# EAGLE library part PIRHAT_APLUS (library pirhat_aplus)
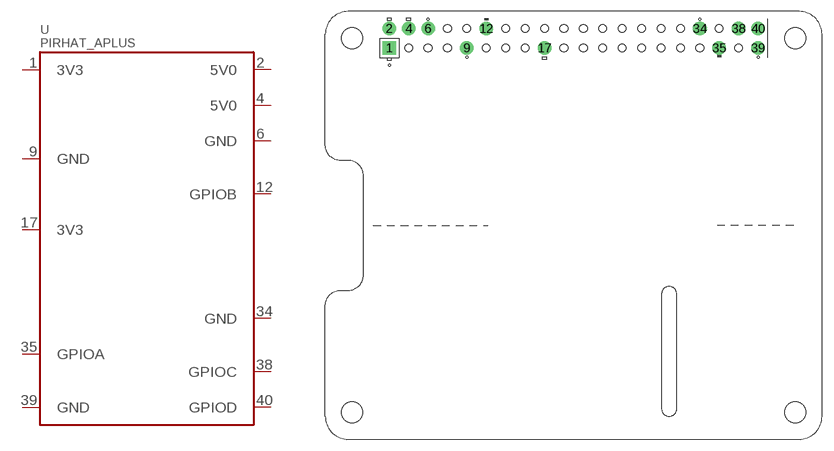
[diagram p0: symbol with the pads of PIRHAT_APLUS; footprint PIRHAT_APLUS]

Designator prefix -

## PIRHAT_APLUS  [PIRHAT_APLUS]
1  3V3  pwr
2  5V0  pwr
4  5V0  pwr
6  GND  sup
9  GND  sup
12  GPIOB
17  3V3  pwr
34  GND  sup
35  GPIOA
38  GPIOC
39  GND  sup
40  GPIOD

## Footprint PIRHAT_APLUS (pad centres in mm)
Raspberry Pi Zero W IR Hat, full outline with position of big connectors & drill holes
drill 1 pad 1.778 square: 1 8.37,51.235
drill 1 pad 1.778: 2 8.37,53.775; 4 10.91,53.775; 6 13.45,53.775; 9 18.53,51.235; 12 21.07,53.775; 17 28.69,51.235; 34 49.01,53.775; 35 51.55,51.235; 38 54.09,53.775; 39 56.63,51.235; 40 56.63,53.775
hole 1 at 54.09,51.235
hole 1 at 51.55,53.775
hole 1 at 31.23,51.235
hole 1 at 26.15,51.235
hole 1 at 15.99,53.775
hole 1 at 49.01,51.235
hole 1 at 23.61,51.235
hole 1 at 15.99,51.235
hole 1 at 13.45,51.235
hole 1 at 10.91,51.235
hole 1 at 21.07,51.235
hole 1 at 23.61,53.775
hole 1 at 28.69,53.775
hole 1 at 31.23,53.775
hole 1 at 26.15,53.775
hole 1 at 18.53,53.775
hole 2.75 at 3.5,3.505
hole 2.75 at 3.5,52.505
hole 2.75 at 61.5,3.505
hole 2.75 at 61.5,52.505
hole 1 at 33.77,51.235
hole 1 at 33.77,53.775
hole 1 at 36.31,53.775
hole 1 at 36.31,51.235
hole 1 at 38.85,53.775
hole 1 at 38.85,51.235
hole 1 at 41.39,53.775
hole 1 at 41.39,51.235
hole 1 at 43.93,53.775
hole 1 at 43.93,51.235
hole 1 at 46.47,53.775
hole 1 at 46.47,51.235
